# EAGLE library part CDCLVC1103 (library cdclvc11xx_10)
CDCLVC1103 3.3V and 2.5V LVCMOS High-Performance Clock Buffer - 1:3 Fan-out Source: http://www.ti.com/lit/ds/symlink/cdclvc1103.pdf
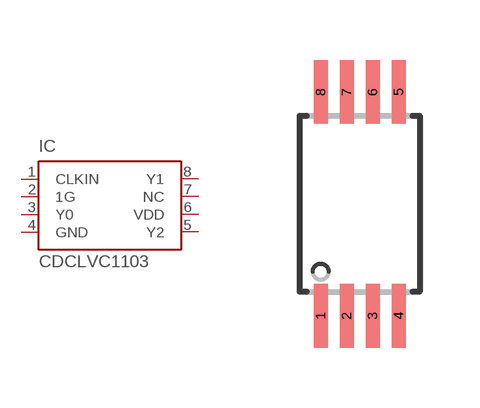
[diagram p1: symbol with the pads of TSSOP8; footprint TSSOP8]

Designator prefix IC

## CDCLVC1103PW (MF: Texas Instruments; MPN: CDCLVC1103; OC_FARNELL: unknown; OC_NEWARK: 79R7908)  [TSSOP8]
1  CLKIN  in
2  1G  in
3  Y0  out
4  GND  pwr
5  Y2  out
6  VDD  pwr
7  NC  nc
8  Y1  out

## Footprint TSSOP8 (pad centres in mm)
TSSOP-8 Plastic Thin Srink Small Outline (PW) Source: http://www.ti.com/lit/ds/symlink/cdclvc1102.pdf
smd 0.35 x 1.6: 1 -0.975,-2.8; 2 -0.325,-2.8; 3 0.325,-2.8; 4 0.975,-2.8; 5 0.975,2.8; 6 0.325,2.8; 7 -0.325,2.8; 8 -0.975,2.8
